|   IBIS model for TI 66ak2h06_12 DSP
[IBIS Ver]   5.0
[Disclaimer]   Please be aware that in the absence of a written agreement
|   Texas Instruments(TI) assumes no liability for:
|   (1) The accuracy of the IBIS models provided to your company,
|   however, the IBIS model is compliant to industry standard
|   IQ Level 2a.  Refer to IBIS Quality Section below for
|   for full details.
|   (2) The proper functioning of these Models in your design
|   or for any resulting applications
|   (3) Infringement of patents, copyrights or intellectual
|   property rights resulting from your use of these
|   models.
|   TI provides IBIS Models as a service to our customers and
|   therefore reserves the right to limit distribution of the
|   Models.  The information is subject to change without notice.
[File Name]  66ak2h06_12_r1p4.ibs
[File Rev]   1.4
[Date]   25 August 2014
[Source]   Texas Instruments Incorporated
[Copyright]   Property of Texas Instruments Incorporated.
|   Unauthorized reproduction and/or distribution is strictly.
|   prohibited.
|   This product is protected under copyright law and trade
|   secret law as an unpublished work.
|   Created 2012,(C) Copyright 1999-2012,
|   Texas Instruments Incorporated., All Rights Reserved.
|   These commodities are under the U.S. Government
|   distribution license control. As such,they are not to be
|   re-exported without the prior approval of the U.S.
|   Department of Commerce.
[Notes]
   For SerDes simulations use Texas Instruments IBIS AMI models
   Some IV curves contain Non monotonic data points.
|   Model Generated by R.L.L.
|   **For SerDes simulations use Texas Instruments IBIS AMI models**
|   This IBIS model also supports 66ak2h06 and 66ak2h12
|   Revision History
|   GERNERAL COMMENT: All IBIS Quality Notes below reflect latest release
|   and version of IBIS File
|   Revision 1.4 -- 25 August 2014  [Formal Updated Release]
|   -Added the [Series Pin Mapping] to assign termination.
|   Revision 1.3 -- 20 August 2014
|   -Updated the signals names to match the data manual
|   Revision 1.2 -- 23 October 2013  [Formal Updated Release]
|   -Cleaned up syntax
|   Revision 1.1 -- 22 October 2013  [Internal Release Only]
|   -Updated All DDR models
|   -Added models for DDR3L support
|   Revision 1.00--25 September 2013
|   -Formal release
|   -Updated pin names
|   Revision 0.23--29 October 2012
|   -updated device nomenclature to match new part numbering scheme
|   Revision 0.22--05 September 2012
|   -Added final packaging and clean up unused IO model selectors
|   Revision 0.21--31 August 2012
|   -Removed models not incorporated in SoC release
|   Revision 0.20--22 August 2012
|   -Added packaging details
|   Revision 0.19--22 August 2012
|   -Preliminary Model Updated
|   -Removed Pkg parasitics to test preliminary release model
|   Revision 0.18--21 August 2012
|   -Preliminary Model Updated
|   Revision 0.17--14 July 2012
|   -Preliminary Model Updated
|   Revision 0.16--14 June 2012
|   -Preliminary Model Updated
|   Revision 0.15--06 June 2012
|   -Preliminary Model Updated
|   Revision 0.14--05 June 2012
|   -Model selector added
|   Revision 0.13--30 May 2012
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[Component] 66ak2hxx
Si_location   Die
Timing_location Die
[Manufacturer] Texas Instruments
|[Package Model] 66ak2hxx
[Package]
|Variable   Typ   Min   Max
R_pkg   1.0013   0.15483   2.0653
L_pkg   2.89689nH  0.94768nH   5.3815nH
C_pkg   1.63791pF  0.87102pF   2.5609pF
[Pin] Signal_name   model_name   | Buffer Name
AM15 RSV185 NC | NC
AM11 RSV099 NC | NC
AW16 RSV161   NC | SERDES
AU16 RSV163   NC | SERDES
AV15 RSV165   NC | SERDES
AW13 RSV167   NC | SERDES
AU13 RSV169   NC | SERDES
AV12 RSV171   NC | SERDES
AW17 RSV162   NC | SERDES
AU17 RSV164   NC | SERDES
AV16 RSV166   NC | SERDES
AW14 RSV168   NC | SERDES
AU14 RSV170   NC | SERDES
AV13 RSV172   NC | SERDES
AP17 RSV173   NC | SERDES
AR16 RSV175   NC | SERDES
AT15 RSV177   NC | SERDES
AP14 RSV179   NC | SERDES
AR13 RSV181   NC | SERDES
AT12 RSV183   NC | SERDES
AP18 RSV174   NC | SERDES
AR17 RSV176   NC | SERDES
AT16 RSV178   NC | SERDES
AP15 RSV180   NC | SERDES
AR14 RSV182   NC | SERDES
AT13 RSV184   NC | SERDES
AL2 ALTCORECLKN iclkrx0p9gh | iclkrx0p9gh
AM2 ALTCORECLKP iclkrx0p9gh | iclkrx0p9gh
B37 ARMCLKN iclkrx0p9gh | iclkrx0p9gh
C37 ARMCLKP iclkrx0p9gh | iclkrx0p9gh
AF11 AVDDA1 POWER | POWER
M20 AVDDA10 POWER | POWER
Y28 AVDDA11 POWER | POWER
AB28 AVDDA12 POWER | POWER
AC28 AVDDA13 POWER | POWER
AD28 AVDDA14 POWER | POWER
AE28 AVDDA15 POWER | POWER
N20 AVDDA2 POWER | POWER
N28 AVDDA3 POWER | POWER
AH29 AVDDA4 POWER | POWER
AG26 AVDDA5 POWER | POWER
P11 AVDDA6 POWER | POWER
M13 AVDDA7 POWER | POWER
M15 AVDDA8 POWER | POWER
M18 AVDDA9 POWER | POWER
AF5 BOOTCOMPLETE bc181540h | bc181540edc50bghypbfbh
AL4 CORECLKSEL ic1815ghypbfbh | ic1815ghypbfbh
F24 CORESEL0 bc181540v | bc181540edc50bghypbfbv
E24 CORESEL1 bc181540v | bc181540edc50bghypbfbv
D24 CORESEL2 bc181540v | bc181540edc50bghypbfbv
G24 CORESEL3 bc181540v | bc181540edc50bghypbfbv
AA10 CVDD POWER | POWER
AA16 CVDD POWER | POWER
AA18 CVDD POWER | POWER
AA20 CVDD POWER | POWER
AA22 CVDD POWER | POWER
AA24 CVDD POWER | POWER
AA26 CVDD POWER | POWER
AA8 CVDD POWER | POWER
AB11 CVDD POWER | POWER
AB15 CVDD POWER | POWER
AB17 CVDD POWER | POWER
AB19 CVDD POWER | POWER
AB21 CVDD POWER | POWER
AB23 CVDD POWER | POWER
AB25 CVDD POWER | POWER
AB27 CVDD POWER | POWER
AB9 CVDD POWER | POWER
AC10 CVDD POWER | POWER
AC12 CVDD POWER | POWER
AC14 CVDD POWER | POWER
AC16 CVDD POWER | POWER
AC20 CVDD POWER | POWER
AC22 CVDD POWER | POWER
AC24 CVDD POWER | POWER
AC26 CVDD POWER | POWER
AC8 CVDD POWER | POWER
AD13 CVDD POWER | POWER
AD15 CVDD POWER | POWER
AD21 CVDD POWER | POWER
AD23 CVDD POWER | POWER
AD25 CVDD POWER | POWER
AD27 CVDD POWER | POWER
AD9 CVDD POWER | POWER
AE10 CVDD POWER | POWER
AE12 CVDD POWER | POWER
AE14 CVDD POWER | POWER
AE16 CVDD POWER | POWER
AE18 CVDD POWER | POWER
AE20 CVDD POWER | POWER
AE22 CVDD POWER | POWER
AE24 CVDD POWER | POWER
AE26 CVDD POWER | POWER
AE8 CVDD POWER | POWER
AF25 CVDD POWER | POWER
AF27 CVDD POWER | POWER
AF9 CVDD POWER | POWER
AG10 CVDD POWER | POWER
AG28 CVDD POWER | POWER
AG8 CVDD POWER | POWER
AH27 CVDD POWER | POWER
AH9 CVDD POWER | POWER
AJ10 CVDD POWER | POWER
AJ28 CVDD POWER | POWER
AJ8 CVDD POWER | POWER
AK29 CVDD POWER | POWER
AK7 CVDD POWER | POWER
AK9 CVDD POWER | POWER
AL30 CVDD POWER | POWER
AL6 CVDD POWER | POWER
AL8 CVDD POWER | POWER
AM31 CVDD POWER | POWER
AM5 CVDD POWER | POWER
L6 CVDD POWER | POWER
M25 CVDD POWER | POWER
M7 CVDD POWER | POWER
M9 CVDD POWER | POWER
N10 CVDD POWER | POWER
N12 CVDD POWER | POWER
N14 CVDD POWER | POWER
N16 CVDD POWER | POWER
N18 CVDD POWER | POWER
N22 CVDD POWER | POWER
N6 CVDD POWER | POWER
N8 CVDD POWER | POWER
P13 CVDD POWER | POWER
P15 CVDD POWER | POWER
P17 CVDD POWER | POWER
P19 CVDD POWER | POWER
P21 CVDD POWER | POWER
P27 CVDD POWER | POWER
P7 CVDD POWER | POWER
P9 CVDD POWER | POWER
R10 CVDD POWER | POWER
R12 CVDD POWER | POWER
R14 CVDD POWER | POWER
R16 CVDD POWER | POWER
R18 CVDD POWER | POWER
R20 CVDD POWER | POWER
R8 CVDD POWER | POWER
T11 CVDD POWER | POWER
T15 CVDD POWER | POWER
T17 CVDD POWER | POWER
T19 CVDD POWER | POWER
T27 CVDD POWER | POWER
T9 CVDD POWER | POWER
U10 CVDD POWER | POWER
U12 CVDD POWER | POWER
U18 CVDD POWER | POWER
U8 CVDD POWER | POWER
V15 CVDD POWER | POWER
V19 CVDD POWER | POWER
V27 CVDD POWER | POWER
V9 CVDD POWER | POWER
W10 CVDD POWER | POWER
W12 CVDD POWER | POWER
W14 CVDD POWER | POWER
W18 CVDD POWER | POWER
W20 CVDD POWER | POWER
W8 CVDD POWER | POWER
Y15 CVDD POWER | POWER
Y17 CVDD POWER | POWER
Y19 CVDD POWER | POWER
Y21 CVDD POWER | POWER
Y23 CVDD POWER | POWER
Y25 CVDD POWER | POWER
Y27 CVDD POWER | POWER
Y9 CVDD POWER | POWER
AC18 CVDD1 POWER | POWER
AD17 CVDD1 POWER | POWER
AD19 CVDD1 POWER | POWER
T13 CVDD1 POWER | POWER
T21 CVDD1 POWER | POWER
U14 CVDD1 POWER | POWER
U16 CVDD1 POWER | POWER
U20 CVDD1 POWER | POWER
V13 CVDD1 POWER | POWER
V17 CVDD1 POWER | POWER
V21 CVDD1 POWER | POWER
W16 CVDD1 POWER | POWER
AF13 VDDALV POWER | POWER
AF15 VDDALV POWER | POWER
AF17 VDDALV POWER | POWER
AF19 VDDALV POWER | POWER
AF21 VDDALV POWER | POWER
AF23 VDDALV POWER | POWER
AG12 VDDALV POWER | POWER
AG14 VDDALV POWER | POWER
AG16 VDDALV POWER | POWER
AG18 VDDALV POWER | POWER
AG20 VDDALV POWER | POWER
AG22 VDDALV POWER | POWER
AH11 VDDALV POWER | POWER
AH13 VDDALV POWER | POWER
AH15 VDDALV POWER | POWER
AH17 VDDALV POWER | POWER
AH19 VDDALV POWER | POWER
AH21 VDDALV POWER | POWER
AH23 VDDALV POWER | POWER
AH25 VDDALV POWER | POWER
AJ12 VDDALV POWER | POWER
AJ14 VDDALV POWER | POWER
AJ16 VDDALV POWER | POWER
AJ18 VDDALV POWER | POWER
AJ20 VDDALV POWER | POWER
AJ22 VDDALV POWER | POWER
AJ24 VDDALV POWER | POWER
H31 CVDD POWER | POWER
J30 CVDD POWER | POWER
K29 CVDD POWER | POWER
L28 CVDD POWER | POWER
M27 CVDD POWER | POWER
N24 CVDD POWER | POWER
N26 CVDD POWER | POWER
P23 CVDD POWER | POWER
P25 CVDD POWER | POWER
R24 CVDD POWER | POWER
R26 CVDD POWER | POWER
T23 CVDD POWER | POWER
T25 CVDD POWER | POWER
U24 CVDD POWER | POWER
U26 CVDD POWER | POWER
V23 CVDD POWER | POWER
V25 CVDD POWER | POWER
W24 CVDD POWER | POWER
W26 CVDD POWER | POWER
R22 CVDDT1 POWER | POWER
U22 CVDDT1 POWER | POWER
W22 CVDDT1 POWER | POWER
E8 DDR3AA00 ACC_OUT | SNPS_D3F_PDDRIO_NS
G9 DDR3AA01 ACC_OUT | SNPS_D3F_PDDRIO_NS
G8 DDR3AA02 ACC_OUT | SNPS_D3F_PDDRIO_NS
G10 DDR3AA03 ACC_OUT | SNPS_D3F_PDDRIO_NS
F9 DDR3AA04 ACC_OUT | SNPS_D3F_PDDRIO_NS
F8 DDR3AA05 ACC_OUT | SNPS_D3F_PDDRIO_NS
C9 DDR3AA06 ACC_OUT | SNPS_D3F_PDDRIO_NS
D9 DDR3AA07 ACC_OUT | SNPS_D3F_PDDRIO_NS
B9 DDR3AA08 ACC_OUT | SNPS_D3F_PDDRIO_NS
D8 DDR3AA09 ACC_OUT | SNPS_D3F_PDDRIO_NS
F10 DDR3AA10 ACC_OUT | SNPS_D3F_PDDRIO_NS
A9 DDR3AA11 ACC_OUT | SNPS_D3F_PDDRIO_NS
E10 DDR3AA12 ACC_OUT | SNPS_D3F_PDDRIO_NS
A10 DDR3AA13 ACC_OUT | SNPS_D3F_PDDRIO_NS
B10 DDR3AA14 ACC_OUT | SNPS_D3F_PDDRIO_NS
D10 DDR3AA15 ACC_OUT | SNPS_D3F_PDDRIO_NS
B11 DDR3ABA0 ACC_OUT | SNPS_D3F_PDDRIO_NS
C11 DDR3ABA1 ACC_OUT | SNPS_D3F_PDDRIO_NS
G11 DDR3ABA2 ACC_OUT | SNPS_D3F_PDDRIO_NS
C13 DDR3ACAS ACC_OUT | SNPS_D3F_PDDRIO_NS
A16 DDR3ACB00 DQ | SNPS_D3F_PDDRIO_NS
C15 DDR3ACB01 DQ | SNPS_D3F_PDDRIO_NS
B16 DDR3ACB02 DQ | SNPS_D3F_PDDRIO_NS
F15 DDR3ACB03 DQ | SNPS_D3F_PDDRIO_NS
D15 DDR3ACB04 DQ | SNPS_D3F_PDDRIO_NS
F14 DDR3ACB05 DQ | SNPS_D3F_PDDRIO_NS
D14 DDR3ACB06 DQ | SNPS_D3F_PDDRIO_NS
G15 DDR3ACB07 DQ | SNPS_D3F_PDDRIO_NS
D11 DDR3ACE0 ACC_OUT | SNPS_D3F_PDDRIO_NS
F11 DDR3ACE1 ACC_OUT | SNPS_D3F_PDDRIO_NS
G12 DDR3ACKE0 ACC_OUT | SNPS_D3F_PDDRIO_NS
A11 DDR3ACKE1 ACC_OUT | SNPS_D3F_PDDRIO_NS
A25 DDR3ACLKN iclkrx0p9gv | iclkrx0p9gv
B12 DDR3ACLKOUTN0 CLK_OUT | SNPS_D3F_PDDRIO_NS
B13 DDR3ACLKOUTN1 CLK_OUT | SNPS_D3F_PDDRIO_NS
A12 DDR3ACLKOUTP0 CLK_OUT | SNPS_D3F_PDDRIO_NS
A13 DDR3ACLKOUTP1 CLK_OUT | SNPS_D3F_PDDRIO_NS
B25 DDR3ACLKP iclkrx0p9gv | iclkrx0p9gv
G1 DDR3AD00 DQ | SNPS_D3F_PDDRIO_NS
H2 DDR3AD01 DQ | SNPS_D3F_PDDRIO_NS
F1 DDR3AD02 DQ | SNPS_D3F_PDDRIO_NS
G2 DDR3AD03 DQ | SNPS_D3F_PDDRIO_NS
H1 DDR3AD04 DQ | SNPS_D3F_PDDRIO_NS
E2 DDR3AD05 DQ | SNPS_D3F_PDDRIO_NS
F2 DDR3AD06 DQ | SNPS_D3F_PDDRIO_NS
D2 DDR3AD07 DQ | SNPS_D3F_PDDRIO_NS
E4 DDR3AD08 DQ | SNPS_D3F_PDDRIO_NS
F4 DDR3AD09 DQ | SNPS_D3F_PDDRIO_NS
G3 DDR3AD10 DQ | SNPS_D3F_PDDRIO_NS
A4 DDR3AD11 DQ | SNPS_D3F_PDDRIO_NS
B4 DDR3AD12 DQ | SNPS_D3F_PDDRIO_NS
H3 DDR3AD13 DQ | SNPS_D3F_PDDRIO_NS
D3 DDR3AD14 DQ | SNPS_D3F_PDDRIO_NS
D4 DDR3AD15 DQ | SNPS_D3F_PDDRIO_NS
G4 DDR3AD16 DQ | SNPS_D3F_PDDRIO_NS
H5 DDR3AD17 DQ | SNPS_D3F_PDDRIO_NS
D5 DDR3AD18 DQ | SNPS_D3F_PDDRIO_NS
F5 DDR3AD19 DQ | SNPS_D3F_PDDRIO_NS
G5 DDR3AD20 DQ | SNPS_D3F_PDDRIO_NS
D6 DDR3AD21 DQ | SNPS_D3F_PDDRIO_NS
C5 DDR3AD22 DQ | SNPS_D3F_PDDRIO_NS
B6 DDR3AD23 DQ | SNPS_D3F_PDDRIO_NS
C7 DDR3AD24 DQ | SNPS_D3F_PDDRIO_NS
F7 DDR3AD25 DQ | SNPS_D3F_PDDRIO_NS
F6 DDR3AD26 DQ | SNPS_D3F_PDDRIO_NS
A8 DDR3AD27 DQ | SNPS_D3F_PDDRIO_NS
B8 DDR3AD28 DQ | SNPS_D3F_PDDRIO_NS
G6 DDR3AD29 DQ | SNPS_D3F_PDDRIO_NS
G7 DDR3AD30 DQ | SNPS_D3F_PDDRIO_NS
D7 DDR3AD31 DQ | SNPS_D3F_PDDRIO_NS
E16 DDR3AD32 DQ | SNPS_D3F_PDDRIO_NS
G16 DDR3AD33 DQ | SNPS_D3F_PDDRIO_NS
F16 DDR3AD34 DQ | SNPS_D3F_PDDRIO_NS
G17 DDR3AD35 DQ | SNPS_D3F_PDDRIO_NS
D16 DDR3AD36 DQ | SNPS_D3F_PDDRIO_NS
D17 DDR3AD37 DQ | SNPS_D3F_PDDRIO_NS
F17 DDR3AD38 DQ | SNPS_D3F_PDDRIO_NS
E18 DDR3AD39 DQ | SNPS_D3F_PDDRIO_NS
C19 DDR3AD40 DQ | SNPS_D3F_PDDRIO_NS
D19 DDR3AD41 DQ | SNPS_D3F_PDDRIO_NS
G18 DDR3AD42 DQ | SNPS_D3F_PDDRIO_NS
F19 DDR3AD43 DQ | SNPS_D3F_PDDRIO_NS
G19 DDR3AD44 DQ | SNPS_D3F_PDDRIO_NS
B18 DDR3AD45 DQ | SNPS_D3F_PDDRIO_NS
D18 DDR3AD46 DQ | SNPS_D3F_PDDRIO_NS
F18 DDR3AD47 DQ | SNPS_D3F_PDDRIO_NS
A20 DDR3AD48 DQ | SNPS_D3F_PDDRIO_NS
B20 DDR3AD49 DQ | SNPS_D3F_PDDRIO_NS
D20 DDR3AD50 DQ | SNPS_D3F_PDDRIO_NS
G20 DDR3AD51 DQ | SNPS_D3F_PDDRIO_NS
C21 DDR3AD52 DQ | SNPS_D3F_PDDRIO_NS
E20 DDR3AD53 DQ | SNPS_D3F_PDDRIO_NS
F20 DDR3AD54 DQ | SNPS_D3F_PDDRIO_NS
G21 DDR3AD55 DQ | SNPS_D3F_PDDRIO_NS
C23 DDR3AD56 DQ | SNPS_D3F_PDDRIO_NS
G22 DDR3AD57 DQ | SNPS_D3F_PDDRIO_NS
D23 DDR3AD58 DQ | SNPS_D3F_PDDRIO_NS
F22 DDR3AD59 DQ | SNPS_D3F_PDDRIO_NS
E22 DDR3AD60 DQ | SNPS_D3F_PDDRIO_NS
B22 DDR3AD61 DQ | SNPS_D3F_PDDRIO_NS
F21 DDR3AD62 DQ | SNPS_D3F_PDDRIO_NS
D22 DDR3AD63 DQ | SNPS_D3F_PDDRIO_NS
C2 DDR3ADQM0 DM | SNPS_D3F_PDDRIO_NS
F3 DDR3ADQM1 DM | SNPS_D3F_PDDRIO_NS
A6 DDR3ADQM2 DM | SNPS_D3F_PDDRIO_NS
E6 DDR3ADQM3 DM | SNPS_D3F_PDDRIO_NS
C17 DDR3ADQM4 DM | SNPS_D3F_PDDRIO_NS
A18 DDR3ADQM5 DM | SNPS_D3F_PDDRIO_NS
D21 DDR3ADQM6 DM | SNPS_D3F_PDDRIO_NS
A22 DDR3ADQM7 DM | SNPS_D3F_PDDRIO_NS
E14 DDR3ADQM8 DM | SNPS_D3F_PDDRIO_NS
D1 DDR3ADQS0N DQS | SNPS_D3F_PDIFF_NS
E1 DDR3ADQS0P DQS | SNPS_D3F_PDIFF_NS
C3 DDR3ADQS1N DQS | SNPS_D3F_PDIFF_NS
B3 DDR3ADQS1P DQS | SNPS_D3F_PDIFF_NS
B5 DDR3ADQS2N DQS | SNPS_D3F_PDIFF_NS
A5 DDR3ADQS2P DQS | SNPS_D3F_PDIFF_NS
A7 DDR3ADQS3N DQS | SNPS_D3F_PDIFF_NS
B7 DDR3ADQS3P DQS | SNPS_D3F_PDIFF_NS
B17 DDR3ADQS4N DQS | SNPS_D3F_PDIFF_NS
A17 DDR3ADQS4P DQS | SNPS_D3F_PDIFF_NS
A19 DDR3ADQS5N DQS | SNPS_D3F_PDIFF_NS
B19 DDR3ADQS5P DQS | SNPS_D3F_PDIFF_NS
B21 DDR3ADQS6N DQS | SNPS_D3F_PDIFF_NS
A21 DDR3ADQS6P DQS | SNPS_D3F_PDIFF_NS
B23 DDR3ADQS7N DQS | SNPS_D3F_PDIFF_NS
A23 DDR3ADQS7P DQS | SNPS_D3F_PDIFF_NS
A15 DDR3ADQS8N DQS | SNPS_D3F_PDIFF_NS
B15 DDR3ADQS8P DQS | SNPS_D3F_PDIFF_NS
E12 DDR3AODT0 ACC_OUT | SNPS_D3F_PDDRIO_NS
G13 DDR3AODT1 ACC_OUT | SNPS_D3F_PDDRIO_NS
A14 DDR3ARAS ACC_OUT | SNPS_D3F_PDDRIO_NS
B14 DDR3ARESET ACC_OUT | SNPS_D3F_PDDRIO_NS
H16 DDR3ARZQ0 NC | SNPS_D3F_PZQ_NS
H10 DDR3ARZQ1 NC | SNPS_D3F_PZQ_NS
H22 DDR3ARZQ2 NC | SNPS_D3F_PZQ_NS
G14 DDR3AVREFSSTL POWER | POWER
F12 DDR3AWE ACC_OUT | SNPS_D3F_PDDRIO_NS
AA32 DDR3BA00 ACC_OUT | SNPS_D3F_PDDRIO_NS
W33 DDR3BA01 ACC_OUT | SNPS_D3F_PDDRIO_NS
W32 DDR3BA02 ACC_OUT | SNPS_D3F_PDDRIO_NS
Y34 DDR3BA03 ACC_OUT | SNPS_D3F_PDDRIO_NS
W34 DDR3BA04 ACC_OUT | SNPS_D3F_PDDRIO_NS
V34 DDR3BA05 ACC_OUT | SNPS_D3F_PDDRIO_NS
W36 DDR3BA06 ACC_OUT | SNPS_D3F_PDDRIO_NS
W37 DDR3BA07 ACC_OUT | SNPS_D3F_PDDRIO_NS
AA33 DDR3BA08 ACC_OUT | SNPS_D3F_PDDRIO_NS
Y32 DDR3BA09 ACC_OUT | SNPS_D3F_PDDRIO_NS
Y38 DDR3BA10 ACC_OUT | SNPS_D3F_PDDRIO_NS
AA39 DDR3BA11 ACC_OUT | SNPS_D3F_PDDRIO_NS
Y35 DDR3BA12 ACC_OUT | SNPS_D3F_PDDRIO_NS
Y39 DDR3BA13 ACC_OUT | SNPS_D3F_PDDRIO_NS
AA38 DDR3BA14 ACC_OUT | SNPS_D3F_PDDRIO_NS
Y36 DDR3BA15 ACC_OUT | SNPS_D3F_PDDRIO_NS
AA37 DDR3BBA0 ACC_OUT | SNPS_D3F_PDDRIO_NS
AA34 DDR3BBA1 ACC_OUT | SNPS_D3F_PDDRIO_NS
AB35 DDR3BBA2 ACC_OUT | SNPS_D3F_PDDRIO_NS
AC36 DDR3BCAS ACC_OUT | SNPS_D3F_PDDRIO_NS
AF32 DDR3BCB00 DQ | SNPS_D3F_PDDRIO_NS
AF34 DDR3BCB01 DQ | SNPS_D3F_PDDRIO_NS
AE32 DDR3BCB02 DQ | SNPS_D3F_PDDRIO_NS
AF35 DDR3BCB03 DQ | SNPS_D3F_PDDRIO_NS
AE33 DDR3BCB04 DQ | SNPS_D3F_PDDRIO_NS
AE36 DDR3BCB05 DQ | SNPS_D3F_PDDRIO_NS
AD36 DDR3BCB06 DQ | SNPS_D3F_PDDRIO_NS
AE34 DDR3BCB07 DQ | SNPS_D3F_PDDRIO_NS
AB34 DDR3BCE0 ACC_OUT | SNPS_D3F_PDDRIO_NS
AA36 DDR3BCE1 ACC_OUT | SNPS_D3F_PDDRIO_NS
AB39 DDR3BCKE0 ACC_OUT | SNPS_D3F_PDDRIO_NS
AB38 DDR3BCKE1 ACC_OUT | SNPS_D3F_PDDRIO_NS
AR39 DDR3BCLKN iclkrx0p9gv | iclkrx0p9gv
AD39 DDR3BCLKOUTN0 CLK_OUT | SNPS_D3F_PDDRIO_NS
AC38 DDR3BCLKOUTN1 CLK_OUT | SNPS_D3F_PDDRIO_NS
AD38 DDR3BCLKOUTP0 CLK_OUT | SNPS_D3F_PDDRIO_NS
AC39 DDR3BCLKOUTP1 CLK_OUT | SNPS_D3F_PDDRIO_NS
AR38 DDR3BCLKP iclkrx0p9gv | iclkrx0p9gv
L38 DDR3BD00 DQ | SNPS_D3F_PDDRIO_NS
N34 DDR3BD01 DQ | SNPS_D3F_PDDRIO_NS
M37 DDR3BD02 DQ | SNPS_D3F_PDDRIO_NS
L39 DDR3BD03 DQ | SNPS_D3F_PDDRIO_NS
N33 DDR3BD04 DQ | SNPS_D3F_PDDRIO_NS
N37 DDR3BD05 DQ | SNPS_D3F_PDDRIO_NS
N36 DDR3BD06 DQ | SNPS_D3F_PDDRIO_NS
N38 DDR3BD07 DQ | SNPS_D3F_PDDRIO_NS
T32 DDR3BD08 DQ | SNPS_D3F_PDDRIO_NS
R32 DDR3BD09 DQ | SNPS_D3F_PDDRIO_NS
P35 DDR3BD10 DQ | SNPS_D3F_PDDRIO_NS
R39 DDR3BD11 DQ | SNPS_D3F_PDDRIO_NS
R38 DDR3BD12 DQ | SNPS_D3F_PDDRIO_NS
N32 DDR3BD13 DQ | SNPS_D3F_PDDRIO_NS
R33 DDR3BD14 DQ | SNPS_D3F_PDDRIO_NS
P36 DDR3BD15 DQ | SNPS_D3F_PDDRIO_NS
T34 DDR3BD16 DQ | SNPS_D3F_PDDRIO_NS
R34 DDR3BD17 DQ | SNPS_D3F_PDDRIO_NS
T35 DDR3BD18 DQ | SNPS_D3F_PDDRIO_NS
R37 DDR3BD19 DQ | SNPS_D3F_PDDRIO_NS
R36 DDR3BD20 DQ | SNPS_D3F_PDDRIO_NS
U37 DDR3BD21 DQ | SNPS_D3F_PDDRIO_NS
T36 DDR3BD22 DQ | SNPS_D3F_PDDRIO_NS
U38 DDR3BD23 DQ | SNPS_D3F_PDDRIO_NS
V35 DDR3BD24 DQ | SNPS_D3F_PDDRIO_NS
U36 DDR3BD25 DQ | SNPS_D3F_PDDRIO_NS
U34 DDR3BD26 DQ | SNPS_D3F_PDDRIO_NS
W38 DDR3BD27 DQ | SNPS_D3F_PDDRIO_NS
W39 DDR3BD28 DQ | SNPS_D3F_PDDRIO_NS
U33 DDR3BD29 DQ | SNPS_D3F_PDDRIO_NS
V32 DDR3BD30 DQ | SNPS_D3F_PDDRIO_NS
V36 DDR3BD31 DQ | SNPS_D3F_PDDRIO_NS
AG37 DDR3BD32 DQ | SNPS_D3F_PDDRIO_NS
AF36 DDR3BD33 DQ | SNPS_D3F_PDDRIO_NS
AG38 DDR3BD34 DQ | SNPS_D3F_PDDRIO_NS
AG34 DDR3BD35 DQ | SNPS_D3F_PDDRIO_NS
AG36 DDR3BD36 DQ | SNPS_D3F_PDDRIO_NS
AH34 DDR3BD37 DQ | SNPS_D3F_PDDRIO_NS
AH35 DDR3BD38 DQ | SNPS_D3F_PDDRIO_NS
AG32 DDR3BD39 DQ | SNPS_D3F_PDDRIO_NS
AH32 DDR3BD40 DQ | SNPS_D3F_PDDRIO_NS
AJ33 DDR3BD41 DQ | SNPS_D3F_PDDRIO_NS
AH36 DDR3BD42 DQ | SNPS_D3F_PDDRIO_NS
AJ34 DDR3BD43 DQ | SNPS_D3F_PDDRIO_NS
AJ36 DDR3BD44 DQ | SNPS_D3F_PDDRIO_NS
AH39 DDR3BD45 DQ | SNPS_D3F_PDDRIO_NS
AH38 DDR3BD46 DQ | SNPS_D3F_PDDRIO_NS
AJ37 DDR3BD47 DQ | SNPS_D3F_PDDRIO_NS
AK39 DDR3BD48 DQ | SNPS_D3F_PDDRIO_NS
AK38 DDR3BD49 DQ | SNPS_D3F_PDDRIO_NS
AK36 DDR3BD50 DQ | SNPS_D3F_PDDRIO_NS
AK35 DDR3BD51 DQ | SNPS_D3F_PDDRIO_NS
AL34 DDR3BD52 DQ | SNPS_D3F_PDDRIO_NS
AL36 DDR3BD53 DQ | SNPS_D3F_PDDRIO_NS
AL37 DDR3BD54 DQ | SNPS_D3F_PDDRIO_NS
AL33 DDR3BD55 DQ | SNPS_D3F_PDDRIO_NS
AN34 DDR3BD56 DQ | SNPS_D3F_PDDRIO_NS
AN36 DDR3BD57 DQ | SNPS_D3F_PDDRIO_NS
AN33 DDR3BD58 DQ | SNPS_D3F_PDDRIO_NS
AM34 DDR3BD59 DQ | SNPS_D3F_PDDRIO_NS
AM35 DDR3BD60 DQ | SNPS_D3F_PDDRIO_NS
AM38 DDR3BD61 DQ | SNPS_D3F_PDDRIO_NS
AM36 DDR3BD62 DQ | SNPS_D3F_PDDRIO_NS
AN37 DDR3BD63 DQ | SNPS_D3F_PDDRIO_NS
N39 DDR3BDQM0 DM | SNPS_D3F_PDDRIO_NS
P34 DDR3BDQM1 DM | SNPS_D3F_PDDRIO_NS
U39 DDR3BDQM2 DM | SNPS_D3F_PDDRIO_NS
U32 DDR3BDQM3 DM | SNPS_D3F_PDDRIO_NS
AG33 DDR3BDQM4 DM | SNPS_D3F_PDDRIO_NS
AG39 DDR3BDQM5 DM | SNPS_D3F_PDDRIO_NS
AK34 DDR3BDQM6 DM | SNPS_D3F_PDDRIO_NS
AM39 DDR3BDQM7 DM | SNPS_D3F_PDDRIO_NS
AE37 DDR3BDQM8 DM | SNPS_D3F_PDDRIO_NS
M39 DDR3BDQS0N DQS | SNPS_D3F_PDIFF_NS
M38 DDR3BDQS0P DQS | SNPS_D3F_PDIFF_NS
P38 DDR3BDQS1N DQS | SNPS_D3F_PDIFF_NS
P39 DDR3BDQS1P DQS | SNPS_D3F_PDIFF_NS
T38 DDR3BDQS2N DQS | SNPS_D3F_PDIFF_NS
T39 DDR3BDQS2P DQS | SNPS_D3F_PDIFF_NS
V38 DDR3BDQS3N DQS | SNPS_D3F_PDIFF_NS
V39 DDR3BDQS3P DQS | SNPS_D3F_PDIFF_NS
AF39 DDR3BDQS4N DQS | SNPS_D3F_PDIFF_NS
AF38 DDR3BDQS4P DQS | SNPS_D3F_PDIFF_NS
AJ38 DDR3BDQS5N DQS | SNPS_D3F_PDIFF_NS
AJ39 DDR3BDQS5P DQS | SNPS_D3F_PDIFF_NS
AL38 DDR3BDQS6N DQS | SNPS_D3F_PDIFF_NS
AL39 DDR3BDQS6P DQS | SNPS_D3F_PDIFF_NS
AN39 DDR3BDQS7N DQS | SNPS_D3F_PDIFF_NS
AN38 DDR3BDQS7P DQS | SNPS_D3F_PDIFF_NS
AE38 DDR3BDQS8N DQS | SNPS_D3F_PDIFF_NS
AE39 DDR3BDQS8P DQS | SNPS_D3F_PDIFF_NS
AC33 DDR3BODT0 ACC_OUT   | SNPS_D3F_PDDRIO_NS
AD34 DDR3BODT1 ACC_OUT   | SNPS_D3F_PDDRIO_NS
AD32 DDR3BRAS ACC_OUT   | SNPS_D3F_PDDRIO_NS
AC32 DDR3BRESET ACC_OUT | SNPS_D3F_PDDRIO_NS
AA31 DDR3BRZQ0 NC | SNPS_D3F_PZQ_NS
P32 DDR3BRZQ1 NC  | SNPS_D3F_PZQ_NS
AK32 DDR3BRZQ2 NC | SNPS_D3F_PZQ_NS
AC31 DDR3BVREFSSTL POWER | POWER
AC37 DDR3BWE ACC_OUT | SNPS_D3F_PDDRIO_NS
AA28 DVDD15 POWER | POWER
AA30 DVDD15 POWER | POWER
AB29 DVDD15 POWER | POWER
AB31 DVDD15 POWER | POWER
AC30 DVDD15 POWER | POWER
AD29 DVDD15 POWER | POWER
AD31 DVDD15 POWER | POWER
AE30 DVDD15 POWER | POWER
AF29 DVDD15 POWER | POWER
AF31 DVDD15 POWER | POWER
AG30 DVDD15 POWER | POWER
AH31 DVDD15 POWER | POWER
AJ30 DVDD15 POWER | POWER
AK31 DVDD15 POWER | POWER
AL32 DVDD15 POWER | POWER
H11 DVDD15 POWER  | POWER
H13 DVDD15 POWER  | POWER
H15 DVDD15 POWER  | POWER
H17 DVDD15 POWER  | POWER
H19 DVDD15 POWER  | POWER
H21 DVDD15 POWER  | POWER
H23 DVDD15 POWER  | POWER
H7 DVDD15 POWER   | POWER
H9 DVDD15 POWER   | POWER
J10 DVDD15 POWER | POWER
J12 DVDD15 POWER | POWER
J14 DVDD15 POWER | POWER
J16 DVDD15 POWER | POWER
J18 DVDD15 POWER | POWER
J20 DVDD15 POWER | POWER
J22 DVDD15 POWER | POWER
J6 DVDD15 POWER  | POWER
J8 DVDD15 POWER  | POWER
K11 DVDD15 POWER | POWER
K13 DVDD15 POWER | POWER
K15 DVDD15 POWER | POWER
K17 DVDD15 POWER | POWER
K19 DVDD15 POWER | POWER
K21 DVDD15 POWER | POWER
K23 DVDD15 POWER | POWER
K7 DVDD15 POWER  | POWER
K9 DVDD15 POWER  | POWER
L10 DVDD15 POWER | POWER
L12 DVDD15 POWER | POWER
L14 DVDD15 POWER | POWER
L16 DVDD15 POWER | POWER
L18 DVDD15 POWER | POWER
L20 DVDD15 POWER | POWER
L32 DVDD15 POWER | POWER
L8 DVDD15 POWER  | POWER
M11 DVDD15 POWER | POWER
M17 DVDD15 POWER | POWER
M19 DVDD15 POWER | POWER
M31 DVDD15 POWER | POWER
P29 DVDD15 POWER | POWER
P31 DVDD15 POWER | POWER
R28 DVDD15 POWER | POWER
R30 DVDD15 POWER | POWER
T29 DVDD15 POWER | POWER
T31 DVDD15 POWER | POWER
U28 DVDD15 POWER | POWER
U30 DVDD15 POWER | POWER
V29 DVDD15 POWER | POWER
V31 DVDD15 POWER | POWER
W28 DVDD15 POWER | POWER
W30 DVDD15 POWER | POWER
Y29 DVDD15 POWER | POWER
Y31 DVDD15 POWER | POWER
AA6 DVDD18 POWER | POWER
AB5 DVDD18 POWER | POWER
AB7 DVDD18 POWER | POWER
AC6 DVDD18 POWER | POWER
AD7 DVDD18 POWER | POWER
AE6 DVDD18 POWER | POWER
AF7 DVDD18 POWER | POWER
AG6 DVDD18 POWER | POWER
AJ26 DVDD18 POWER | POWER
AK27 DVDD18 POWER | POWER
AL26 DVDD18 POWER | POWER
AL28 DVDD18 POWER | POWER
AM27 DVDD18 POWER | POWER
AM29 DVDD18 POWER | POWER
H25 DVDD18 POWER  | POWER
H27 DVDD18 POWER  | POWER
J26 DVDD18 POWER  | POWER
J28 DVDD18 POWER  | POWER
J32 DVDD18 POWER  | POWER
K25 DVDD18 POWER  | POWER
K27 DVDD18 POWER  | POWER
K31 DVDD18 POWER  | POWER
L24 DVDD18 POWER  | POWER
L26 DVDD18 POWER  | POWER
L30 DVDD18 POWER  | POWER
M29 DVDD18 POWER  | POWER
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|********************  DIFF PIN  *******************************
[Diff_pin]   inv_pin vdiff tdelay_typ   tdelay_min  tdelay_max
E1   D1   200mV   NA  NA  NA  || DDR3ADQS0P & DDR3ADQS0N
B3   C3   200mV   NA  NA  NA  || DDR3ADQS1P & DDR3ADQS1N
A5   B5   200mV   NA  NA  NA  || DDR3ADQS2P & DDR3ADQS2N
B7   A7   200mV   NA  NA  NA  || DDR3ADQS3P & DDR3ADQS3N
A17   B17   200mV   NA  NA  NA  || DDR3ADQS4P & DDR3ADQS4N
B19   A19   200mV   NA  NA  NA  || DDR3ADQS5P & DDR3ADQS5N
A21   B21   200mV   NA  NA  NA  || DDR3ADQS6P & DDR3ADQS6N
A23   B23   200mV   NA  NA  NA  || DDR3ADQS7P & DDR3ADQS7N
B15   A15   200mV   NA  NA  NA  || DDR3ADQS8P & DDR3ADQS8N
M38   M39   200mV   NA  NA  NA  || DDR3BDQS0P & DDR3BDQS0N
P39   P38   200mV   NA  NA  NA  || DDR3BDQS1P & DDR3BDQS1N
T39   T38   200mV   NA  NA  NA  || DDR3BDQS2P & DDR3BDQS2N
V39   V38   200mV   NA  NA  NA  || DDR3BDQS3P & DDR3BDQS3N
AF38   AF39   200mV   NA  NA  NA  || DDR3BDQS4P & DDR3BDQS4N
AJ39   AJ38   200mV   NA  NA  NA  || DDR3BDQS5P & DDR3BDQS5N
AL39   AL38   200mV   NA  NA  NA  || DDR3BDQS6P & DDR3BDQS6N
AN38   AN39   200mV   NA  NA  NA  || DDR3BDQS7P & DDR3BDQS7N
AE39   AE38   200mV   NA  NA  NA  || DDR3BDQS8P & DDR3BDQS8N
AL3   AK3   NA   NA  NA  NA  || SYSCLKP & SYSCLKN
AM2   AL2   NA   NA  NA  NA  || ALTCORECLKP & ALTCORECLKN
C37   B37   NA   NA  NA  NA  || ARMCLKP & ARMCLKN
B25   A25   NA   NA  NA  NA  || DDR3ACLKP & DDR3ACLKN
AR38   AR39   NA   NA  NA  NA  || DDR3BCLKP & DDR3BCLKN
AV33   AV34   NA   NA  NA  NA  || PASSCLKP & PASSCLKN
AW31   AW32   NA   NA  NA  NA  || PCIECLKP & PCIECLKN
AW34   AW35   NA   NA  NA  NA  || SRIOSGMIICLKP & SRIOSGMIICLKN
AM1   AL1   NA   NA  NA  NA  || TSREFCLKP & TSREFCLKN
AR2   AP2   NA   NA  NA  NA  || RSV186 & RSV187
AN1   AP1   NA   NA  NA  NA  || TSRXCLKOUT0P & TSRXCLKOUT0N
AN3   AP3   NA   NA  NA  NA  || TSRXCLKOUT1P & TSRXCLKOUT1N
[Series Pin Mapping]   pin_2   model_name
AL2   AM2   s_iclkrx0p9gh   || ALTCORECLKN/P
B37   C37   s_iclkrx0p9gh   || ARMCLKN/P
AK3   AL3   s_iclkrx0p9gh   || SYSCLKN/P
A25   B25   s_iclkrx0p9gv   || DDR3ACLKN/P
AR39   AR38   s_iclkrx0p9gv   || DDR3BCLKN/P
AV34   AV33   s_iclkrx0p9gv   || PASSCLKN/P
AW32   AW31   s_iclkrx0p9gv   || PCIECLKN/P
AW35   AW34   s_iclkrx0p9gv   || SRIOSGMIICLKN/P
|---------------- DDR CLK_OUT IBIS Model -------------------
[Model Selector]   CLK_OUT
|pddrio.ibs   [18 October 2013 revision 0.1]
|renamed PDDRIO_D3FP3_
| ----------- DDR3 CLK_OUT Output Model Selector -----------
PDDRIO_D3FP3_34   DDR3 D3F_PDDRIO cell  Z0=34-Ohm
PDDRIO_D3FP3_40   DDR3 D3F_PDDRIO cell  Z0=40-Ohm
PDDRIO_D3FP3_48   DDR3 D3F_PDDRIO cell  Z0=48-Ohm
| ---------- DDR3L CLK_OUT Output Model Selector -----------
PDDRIO_D3FP3L_34   DDR3L D3F_PDDRIO cell  Z0=34-Ohm
PDDRIO_D3FP3L_40   DDR3L D3F_PDDRIO cell  Z0=40-Ohm
PDDRIO_D3FP3L_48   DDR3L D3F_PDDRIO cell  Z0=48-Ohm
|---------------- DDR ACC_OUT IBIS Model -------------------
[Model Selector]   ACC_OUT
|pddrio.ibs   [18 October 2013 revision 0.1]
|renamed PDDRIO_D3FP3_
| ---------- DDR3 ACC_OUT Output Model Selector ------------
PDDRIO_D3FP3_34   DDR3 D3F_PDDRIO cell  Z0=34-Ohm
PDDRIO_D3FP3_40   DDR3 D3F_PDDRIO cell  Z0=40-Ohm
PDDRIO_D3FP3_48   DDR3 D3F_PDDRIO cell  Z0=48-Ohm
| --------- DDR3L ACC_OUT Output Model Selector ------------
PDDRIO_D3FP3L_34   DDR3L D3F_PDDRIO cell  Z0=34-Ohm
PDDRIO_D3FP3L_40   DDR3L D3F_PDDRIO cell  Z0=40-Ohm
PDDRIO_D3FP3L_48   DDR3L D3F_PDDRIO cell  Z0=48-Ohm
|---------------- DDR DM IBIS Model -------------------
[Model Selector]   DM
|pddrio.ibs   [18 October 2013 revision 0.1]
|renamed PDDRIO_D3FP3_
| ------------- DDR3 DM Output Model Selector --------------
PDDRIO_D3FP3_34   DDR3 D3F_PDDRIO cell  Z0=34-Ohm
PDDRIO_D3FP3_40   DDR3 D3F_PDDRIO cell  Z0=40-Ohm
PDDRIO_D3FP3_48   DDR3 D3F_PDDRIO cell  Z0=48-Ohm
| ------------ DDR3L DM Output Model Selector --------------
PDDRIO_D3FP3L_34   DDR3L D3F_PDDRIO cell  Z0=34-Ohm
PDDRIO_D3FP3L_40   DDR3L D3F_PDDRIO cell  Z0=40-Ohm
PDDRIO_D3FP3L_48   DDR3L D3F_PDDRIO cell  Z0=48-Ohm
| -------------- DDR3 DM Input Model Selector --------------
PDDRIO_D3FP3_ODT120   DDR3 D3F_PDDRIO cell 120-Ohm ODT Receiver
PDDRIO_D3FP3_ODT40   DDR3 D3F_PDDRIO cell 40-Ohm ODT Receiver
PDDRIO_D3FP3_ODT60   DDR3 D3F_PDDRIO cell 60-Ohm ODT Receiver
PDDRIO_D3FP3_ODTOFF   DDR3 D3F_PDDRIO cell ODT off Receiver
| ------------- DDR3L DM Input Model Selector --------------
PDDRIO_D3FP3L_ODT120   DDR3L D3F_PDDRIO cell 120-Ohm ODT Receiver
PDDRIO_D3FP3L_ODT40   DDR3L D3F_PDDRIO cell 40-Ohm ODT Receiver
PDDRIO_D3FP3L_ODT60   DDR3L D3F_PDDRIO cell 60-Ohm ODT Receiver
PDDRIO_D3FP3L_ODTOFF   DDR3L D3F_PDDRIO cell ODT off Receiver
|---------------- DDR DQ IBIS Model -------------------
[Model Selector]   DQ
|pddrio.ibs   [18 October 2013 revision 0.1]
|renamed PDDRIO_D3FP3_
| -------------- DDR3 DQ Output Model Selector --------------
PDDRIO_D3FP3_34   DDR3 D3F_PDDRIO cell  Z0=34-Ohm
PDDRIO_D3FP3_40   DDR3 D3F_PDDRIO cell  Z0=40-Ohm
PDDRIO_D3FP3_48   DDR3 D3F_PDDRIO cell  Z0=48-Ohm
| ------------- DDR3L DQ Output Model Selector --------------
PDDRIO_D3FP3L_34   DDR3L D3F_PDDRIO cell  Z0=34-Ohm
PDDRIO_D3FP3L_40   DDR3L D3F_PDDRIO cell  Z0=40-Ohm
PDDRIO_D3FP3L_48   DDR3L D3F_PDDRIO cell  Z0=48-Ohm
| --------------- DDR3 DQ Input Model Selector --------------
PDDRIO_D3FP3_ODT120   DDR3 D3F_PDDRIO cell 120-Ohm ODT Receiver
PDDRIO_D3FP3_ODT40   DDR3 D3F_PDDRIO cell 40-Ohm ODT Receiver
PDDRIO_D3FP3_ODT60   DDR3 D3F_PDDRIO cell 60-Ohm ODT Receiver
PDDRIO_D3FP3_ODTOFF   DDR3 D3F_PDDRIO cell ODT off Receiver
| -------------- DDR3L DQ Input Model Selector --------------
PDDRIO_D3FP3L_ODT120   DDR3L D3F_PDDRIO cell 120-Ohm ODT Receiver
PDDRIO_D3FP3L_ODT40   DDR3L D3F_PDDRIO cell 40-Ohm ODT Receiver
PDDRIO_D3FP3L_ODT60   DDR3L D3F_PDDRIO cell 60-Ohm ODT Receiver
PDDRIO_D3FP3L_ODTOFF   DDR3L D3F_PDDRIO cell ODT off Receiver
| ----------------- DDR DQS IBIS Model --------------------
[Model Selector]   DQS
|pdiff.ibs   [18 October 2013 revision 0.1]
|renamed PDIFF_D3FP3_
| -------------- DDR3 DQS Input Model Selector ------------
PDIFF_D3FF3_ODT120   DDR3 D3F_PDIFF cell 120-Ohm ODT Receiver
PDIFF_D3FF3_ODT40   DDR3 D3F_PDIFF cell 40-Ohm ODT Receiver
PDIFF_D3FF3_ODT60   DDR3 D3F_PDIFF cell 60-Ohm ODT Receiver
PDIFF_D3FF3_ODTOFF   DDR3 D3F_PDIFF cell ODT off Receiver
| -------------- DDR3L DQS Input Model Selector ------------
PDIFF_D3FF3L_ODT120   DDR3L D3F_PDIFF cell 120-Ohm ODT Receiver
PDIFF_D3FF3L_ODT40   DDR3L D3F_PDIFF cell 40-Ohm ODT Receiver
PDIFF_D3FF3L_ODT60   DDR3L D3F_PDIFF cell 60-Ohm ODT Receiver
PDIFF_D3FF3L_ODTOFF   DDR3L D3F_PDIFF cell ODT off Receiver
| -------------- DDR3 DQS Output Model Selector ------------
PDIFF_D3FF3_34   DDR3 D3F_PDIFF cell  Z0=34-Ohm
PDIFF_D3FF3_40   DDR3 D3F_PDIFF cell  Z0=40-Ohm
PDIFF_D3FF3_48   DDR3 D3F_PDIFF cell  Z0=48-Ohm
| -------------- DDR3L DQS Output Model Selector -----------
PDIFF_D3FF3L_34   DDR3L D3F_PDIFF cell  Z0=34-Ohm
PDIFF_D3FF3L_40   DDR3L D3F_PDIFF cell  Z0=40-Ohm
PDIFF_D3FF3L_48   DDR3L D3F_PDIFF cell  Z0=48-Ohm
|----------------  iclkrx0p9gh IBIS Model --------------
[Model Selector]   iclkrx0p9gh
|iclkrx0p9gh_encmint_0.ibs   [12Feb12 revision 2.0]
|iclkrx0p9gh_encmint_1.ibs   [12Feb12 revision 2.0]
iclkrx0p9gh_encmint_0   Ext. CommMode Used
| When set to zero external common mode used
iclkrx0p9gh_encmint_1   Int. CommMode Used
| When set to one internal common mode used
|----------------  iclkrx0p9gv IBIS Model ---------------
[Model Selector]   iclkrx0p9gv
|iclkrx0p9gv_encmint_0.ibs   [12Feb12 revision 2.0]
|iclkrx0p9gv_encmint_1.ibs   [12Feb12 revision 2.0]
iclkrx0p9gv_encmint_0   Ext. CommMode Used
| When set to zero external common mode used
iclkrx0p9gv_encmint_1   Int. CommMode Used
| When set to one internal common mode used
|----------------  s_iclkrx0p9gh IBIS Model ---------------
[Model Selector]  s_iclkrx0p9gh
s_iclkrx0p9gh_encmint_0   Ext. CommMode Used
s_iclkrx0p9gh_encmint_1   Int. CommMode Used
|----------------  s_iclkrx0p9gv IBIS Model ---------------
[Model Selector]  s_iclkrx0p9gv
s_iclkrx0p9gv_encmint_0   Ext. CommMode Used
s_iclkrx0p9gv_encmint_1   Int. CommMode Used
|----------------  D3F_PZQ_NS IBIS Model -----------
|D3F_PZQ_NS.ibs
|place holder for termination IO buffers
|--------bc181540edc50bghypbfbh IBIS Model -----------
[Model Selector]   bc181540h
|bc181540edc50bghypbfbh.ibs   [23Jan12 revision 1.0]
bc181540h_40CCLASS_1P8  Cell operated at 1.8(nom)
|40CCLASS_1P8; 40C:130MHZ@5PF CLASS IO MODE
bc181540h_WK_PD_ON_1P8  Cell operated at 1.8(nom)
|WK_PD_ON_1P8; INPUT MODE WITH WK_PD_ON
bc181540h_40ECLASS_1P8  Cell operated at 1.8(nom)
|40ECLASS_1P8; 40E:230MHZ@5PF CLASS IO MODE
bc181540h_WK_PU_ON_1P8  Cell operated at 1.8(nom)
|WK_PU_ON_1P8; INPUT MODE WITH WK_PU_ON
bc181540h_40DCLASS_1P8  Cell operated at 1.8(nom)
|40DCLASS_1P8; 40D:200MHZ@5PF CLASS IO MODE
bc181540h_50BCLASS_1P8  Cell operated at 1.8(nom)
|50BCLASS_1P8; 50B:100MHZ@5PF CLASS IO MODE
|------ bc181540edc50bghypbfbv IBIS Model --------
[Model Selector]   bc181540v
|bc181540edc50bghypbfbv.ibs  [23Jan12 revision 1.0]
bc181540v_40CCLASS_1P5  Cell operated at 1.5(nom)
|40CCLASS_1P5; 40C:130MHZ@5PF CLASS IO MODE
bc181540v_WK_PD_ON_1P5  Cell operated at 1.5(nom)
|WK_PD_ON_1P5; INPUT MODE WITH WK_PD_ON
bc181540v_40ECLASS_1P5  Cell operated at 1.5(nom)
|40ECLASS_1P5; 40E:230MHZ@5PF CLASS IO MODE
bc181540v_WK_PU_ON_1P5  Cell operated at 1.5(nom)
|WK_PU_ON_1P5; INPUT MODE WITH WK_PU_ON
bc181540v_40DCLASS_1P5  Cell operated at 1.5(nom)
|40DCLASS_1P5; 40D:200MHZ@5PF CLASS IO MODE
bc181540v_50BCLASS_1P5  Cell operated at 1.5(nom)
|50BCLASS_1P5; 50B:100MHZ@5PF CLASS IO MODE
bc181540v_40CCLASS_1P8  Cell operated at 1.8(nom)
|40CCLASS_1P8; 40C:130MHZ@5PF CLASS IO MODE
bc181540v_WK_PD_ON_1P8  Cell operated at 1.8(nom)
|WK_PD_ON_1P8; INPUT MODE WITH WK_PD_ON
bc181540v_40ECLASS_1P8  Cell operated at 1.8(nom)
|40ECLASS_1P8; 40E:230MHZ@5PF CLASS IO MODE
bc181540v_WK_PU_ON_1P8  Cell operated at 1.8(nom)
|WK_PU_ON_1P8; INPUT MODE WITH WK_PU_ON
bc181540v_40DCLASS_1P8  Cell operated at 1.8(nom)
|40DCLASS_1P8; 40D:200MHZ@5PF CLASS IO MODE
bc181540v_50BCLASS_1P8  Cell operated at 1.8(nom)
|50BCLASS_1P8; 50B:100MHZ@5PF CLASS IO MODE
|--------bi2c1815gfzhsh IBIS Model ----------
[Model Selector]   bi2c1815gfzhsh
|bi2c1815gfzhsh.ibs   [11Jan12 revision 1.0]
bi2c1815h_HS_SLAVE_MODE_1P8  Cell operated at 1.8(nom)
|HS_SLAVE_MODE_1P8; I2C HS SLAVE MODE
bi2c1815h_FAST_STD_1P8  Cell operated at 1.8(nom)
|FAST_STD_1P8; I2C FAST AND STD MODE
bi2c1815h_HS_MASTER_MODE_1P8  Cell operated at 1.8(nom)
|HS_MASTER_MODE_1P8; I2C HS MASTER MODE
|--------- bi2c1815gfzhsv IBIS Model ------------
[Model Selector] bi2c1815gfzhsv
|bi2c1815gfzhsv.ibs   [11Jan12 revision 1.0]
bi2c1815v_HS_SLAVE_MODE_1P8  Cell operated at 1.8(nom)
|HS_SLAVE_MODE_1P8; I2C HS SLAVE MODE
bi2c1815v_FAST_STD_1P8  Cell operated at 1.8(nom)
|FAST_STD_1P8; I2C FAST AND STD MODE
bi2c1815v_HS_MASTER_MODE_1P8  Cell operated at 1.8(nom)
|HS_MASTER_MODE_1P8; I2C HS MASTER MODE
|------- ic1815ghypbfbh IBIS Model ------------
[Model Selector] ic1815ghypbfbh
|ic1815ghypbfbh.ibs   [27Dec11 revision 1.0]
ic1815h_WK_PD_ON_1P8  Cell operated at 1.8(nom)
|WK_PD_ON_1P8; WK_PD_ON
ic1815h_WK_PU_ON_1P8  Cell operated at 1.8(nom)
|WK_PU_ON_1P8; WK_PU_ON
ic1815h_RX_MODE_1P8  Cell operated at 1.8(nom)
|RX_MODE_1P8
|---------------- ic1815ghypbfbv IBIS Model --------
[Model Selector] ic1815ghypbfbv
|ic1815ghypbfbv.ibs   [27Dec11 revision 1.0]
ic1815v_WK_PD_ON_1P8  Cell operated at 1.8(nom)
|WK_PD_ON_1P8; WK_PD_ON
ic1815v_WK_PU_ON_1P8  Cell operated at 1.8(nom)
|WK_PU_ON_1P8; WK_PU_ON
ic1815v_RX_MODE_1P8  Cell operated at 1.8(nom)
|RX_MODE_1P8
|---------------- olvds18gh IBIS Model -----------
[Model Selector] olvds18gh
|olvds18gh.ibs   [30Dec11 revision 1.0]
OLVDS18GH_SUBLVDS_MODE_3MA_100_1P8  Cell operated at 1.8(nom)
|SUBLVDS MODE :3MA OUTPUT CURRENT SETTING WITH 100 OHM INT. TERM.
OLVDS18GH_2MA_200_1P8  Cell operated at 1.8(nom)
|2MA OUTPUT CURRENT SETTING WITH 200 OHM INT. TERM.
OLVDS18GH_4MA_100_1P8  Cell operated at 1.8(nom)
|4MA OUTPUT CURRENT SETTING WITH 100 OHM INT. TERM.
OLVDS18GH_SUBLVDS_MODE_2.5MA_100_1P8  Cell operated at 1.8(nom)
|SUBLVDS MODE : 2.5MA OUTPUT CURRENT SETTING WITH 100 OHM INT. TERM.
OLVDS18GH_3.5MA_100_1P8  Cell operated at 1.8(nom)
|3.5MA OUTPUT CURRENT SETTING WITH 100 OHM INT. TERM.
OLVDS18GH_SUBLVDS_MODE_2.66MA_200_1P8  Cell operated at 1.8(nom)
|SUBLVDS MODE :2.66MA OUTPUT CURRENT SETTING WITH 200 OHM INT. TERM.
OLVDS18GH_SUBLVDS_MODE_2MA_200_1P8  Cell operated at 1.8(nom)
|SUBLVDS MODE :2MA OUTPUT CURRENT SETTING WITH 200 OHM INT. TERM.
OLVDS18GH_4MA_200_1P8  Cell operated at 1.8(nom)
|4MA OUTPUT CURRENT SETTING WITH 200 OHM INT. TERM.
OLVDS18GH_3.33MA_200_1P8  Cell operated at 1.8(nom)
|3.33MA OUTPUT CURRENT SETTING WITH 200 OHM INT. TERM.
OLVDS18GH_SUBLVDS_MODE_4MA_100_1P8  Cell operated at 1.8(nom)
|SUBLVDS MODE :4MA OUTPUT CURRENT SETTING WITH 100 OHM INT. TERM.
OLVDS18GH_SUBLVDS_MODE_3.5MA_100_1P8  Cell operated at 1.8(nom)
|SUBLVDS MODE :3.5MA OUTPUT CURRENT SETTING WITH 100 OHM INT. TERM.
OLVDS18GH_3MA_100_1P8  Cell operated at 1.8(nom)
|3MA OUTPUT CURRENT SETTING WITH 100 OHM INT. TERM.
OLVDS18GH_SUBLVDS_MODE_4MA_200_1P8  Cell operated at 1.8(nom)
|SUBLVDS MODE :4MA OUTPUT CURRENT SETTING WITH 200 OHM INT. TERM.
OLVDS18GH_2.5MA_100_1P8  Cell operated at 1.8(nom)
|2.5MA OUTPUT CURRENT SETTING WITH 100 OHM INT. TERM.
OLVDS18GH_SUBLVDS_MODE_3.33MA_200_1P8  Cell operated at 1.8(nom)
|SUBLVDS MODE :3.33MA OUTPUT CURRENT SETTING WITH 200 OHM INT. TERM.
OLVDS18GH_2.66MA_200_1P8  Cell operated at 1.8(nom)
|   Package Model Definition
[Define Package Model]  66ak2hxx
[Manufacturer]   Texas Instruments Incorporated
[OEM]   Texas Instruments Incorporated
[Description]   66ak2hxx pkg with all signals except AMI
|   file: pgz0877ar-e8_080212
|   file dated: August 30, 2012
[Number Of Pins]   665
[Pin Numbers]
AM16 | 1 BGA-AM16 RSV024
AN16 | 2 BGA-AN16 RSV068
AM15 | 3 BGA-AM15 RSV185
AM14 | 4 BGA-AM14 RSV025
AM11 | 5 BGA-AM11 RSV099
AN10 | 6 BGA-AN10 RSV019
AM9  | 7 BGA-AM9 HYP0REFRES
AW16 | 8 BGA-AW16 RSV161
AW17 | 9 BGA-AW17 RSV162
AV18 | 10 BGA-AV18 RSV061
AU16 | 11 BGA-AU16 RSV163
AU17 | 12 BGA-AU17 RSV164
AV16 | 13 BGA-AV16 RSV166
AV15 | 14 BGA-AV15 RSV165
AW14 | 15 BGA-AW14 RSV168
AW13 | 16 BGA-AW13 RSV167
AU13 | 17 BGA-AU13 RSV169
AU14 | 18 BGA-AU14 RSV170
AV13 | 19 BGA-AV13 RSV172
AV12 | 20 BGA-AV12 RSV171
AW11 | 21 BGA-AW11 HYP0RXP0
AP17 | 22 BGA-AP17 RSV173
AP18 | 23 BGA-AP18 RSV174
AR17 | 24 BGA-AR17 RSV176
AR16 | 25 BGA-AR16 RSV175
AT16 | 26 BGA-AT16 RSV178
AT15 | 27 BGA-AT15 RSV177
AP14 | 28 BGA-AP14 RSV179
AP15 | 29 BGA-AP15 RSV180
AR14 | 30 BGA-AR14 RSV182
AR13 | 31 BGA-AR13 RSV181
AT13 | 32 BGA-AT13 RSV184
AT12 | 33 BGA-AT12 RSV183
AL2  | 34 BGA-AL2 ALTCORECLKN
AM2  | 35 BGA-AM2 ALTCORECLKP
AM4  | 36 BGA-AM4 RSV003
AF5  | 37 BGA-AF5 BOOTCOMPLETE
AG2  | 38 BGA-AG2 HYP1RXFLDAT
AG3  | 39 BGA-AG3 HYP0RXPMDAT
AL4  | 40 BGA-AL4 CORECLKSEL
AK5  | 41 BGA-AK5 RSV012
AK1  | 42 BGA-AK1 SYSCLKOUT
AN4  | 43 BGA-AN4 RSV002
F24  | 44 BGA-F24 CORESEL0
E24  | 45 BGA-E24 CORESEL1
G24  | 46 BGA-G24 CORESEL3
D24  | 47 BGA-D24 CORESEL2
D25  | 48 BGA-D25 SPI2CLK
E8   | 49 BGA-E8 DDR3AA00
F8   | 50 BGA-F8 DDR3AA05
F9   | 51 BGA-F9 DDR3AA04
G9   | 52 BGA-G9 DDR3AA01
G8   | 53 BGA-G8 DDR3AA02
A6   | 54 BGA-A6 DDR3ADQM2
G10  | 55 BGA-G10 DDR3AA03
D8   | 56 BGA-D8 DDR3AA09
C9   | 57 BGA-C9 DDR3AA06
B9   | 58 BGA-B9 DDR3AA08
D9   | 59 BGA-D9 DDR3AA07
A9   | 60 BGA-A9 DDR3AA11
F10  | 61 BGA-F10 DDR3AA10
E10  | 62 BGA-E10 DDR3AA12
D10  | 63 BGA-D10 DDR3AA15
A10  | 64 BGA-A10 DDR3AA13
B10  | 65 BGA-B10 DDR3AA14
F13  | 66 BGA-F13 RSV029
G13  | 67 BGA-G13 DDR3AODT1
D13  | 68 BGA-D13 RSV028
B11  | 69 BGA-B11 DDR3ABA0
C11  | 70 BGA-C11 DDR3ABA1
G12  | 71 BGA-G12 DDR3ACKE0
D11  | 72 BGA-D11 DDR3ACE0
G11  | 73 BGA-G11 DDR3ABA2
F11  | 74 BGA-F11 DDR3ACE1
H10  | 75 BGA-H10 DDR3ARZQ1
C13  | 76 BGA-C13 DDR3ACAS
A11  | 77 BGA-A11 DDR3ACKE1
A16  | 78 BGA-A16 DDR3ACB00
B16  | 79 BGA-B16 DDR3ACB02
C15  | 80 BGA-C15 DDR3ACB01
D15  | 81 BGA-D15 DDR3ACB04
F15  | 82 BGA-F15 DDR3ACB03
F14  | 83 BGA-F14 DDR3ACB05
E14  | 84 BGA-E14 DDR3ADQM8
D14  | 85 BGA-D14 DDR3ACB06
G15  | 86 BGA-G15 DDR3ACB07
F12  | 87 BGA-F12 DDR3AWE
D12  | 88 BGA-D12 RSV027
A25  | 89 BGA-A25 DDR3ACLKN
B25  | 90 BGA-B25 DDR3ACLKP
B24  | 91 BGA-B24 RSV004
B12  | 92 BGA-B12 DDR3ACLKOUTN0
A12  | 93 BGA-A12 DDR3ACLKOUTP0
B13  | 94 BGA-B13 DDR3ACLKOUTN1
A13  | 95 BGA-A13 DDR3ACLKOUTP1
G1   | 96 BGA-G1 DDR3AD00
H2   | 97 BGA-H2 DDR3AD01
G2   | 98 BGA-G2 DDR3AD03
H1   | 99 BGA-H1 DDR3AD04
F1   | 100 BGA-F1 DDR3AD02
E1   | 101 BGA-E1 DDR3ADQS0P
E2   | 102 BGA-E2 DDR3AD05
D2   | 103 BGA-D2 DDR3AD07
F2   | 104 BGA-F2 DDR3AD06
D1   | 105 BGA-D1 DDR3ADQS0N
C2   | 106 BGA-C2 DDR3ADQM0
E4   | 107 BGA-E4 DDR3AD08
D4   | 108 BGA-D4 DDR3AD15
D3   | 109 BGA-D3 DDR3AD14
F4   | 110 BGA-F4 DDR3AD09
G3   | 111 BGA-G3 DDR3AD10
F3   | 112 BGA-F3 DDR3ADQM1
H3   | 113 BGA-H3 DDR3AD13
A4   | 114 BGA-A4 DDR3AD11
B4   | 115 BGA-B4 DDR3AD12
G4   | 116 BGA-G4 DDR3AD16
H5   | 117 BGA-H5 DDR3AD17
G5   | 118 BGA-G5 DDR3AD20
D5   | 119 BGA-D5 DDR3AD18
F5   | 120 BGA-F5 DDR3AD19
A5   | 121 BGA-A5 DDR3ADQS2P
D6   | 122 BGA-D6 DDR3AD21
B6   | 123 BGA-B6 DDR3AD23
C5   | 124 BGA-C5 DDR3AD22
B5   | 125 BGA-B5 DDR3ADQS2N
C7   | 126 BGA-C7 DDR3AD24
D7   | 127 BGA-D7 DDR3AD31
B8   | 128 BGA-B8 DDR3AD28
F7   | 129 BGA-F7 DDR3AD25
G7   | 130 BGA-G7 DDR3AD30
F6   | 131 BGA-F6 DDR3AD26
E6   | 132 BGA-E6 DDR3ADQM3
G6   | 133 BGA-G6 DDR3AD29
A8   | 134 BGA-A8 DDR3AD27
B7   | 135 BGA-B7 DDR3ADQS3P
E16  | 136 BGA-E16 DDR3AD32
D16  | 137 BGA-D16 DDR3AD36
F16  | 138 BGA-F16 DDR3AD34
G16  | 139 BGA-G16 DDR3AD33
G17  | 140 BGA-G17 DDR3AD35
F17  | 141 BGA-F17 DDR3AD38
H16  | 142 BGA-H16 DDR3ARZQ0
D17  | 143 BGA-D17 DDR3AD37
C17  | 144 BGA-C17 DDR3ADQM4
E18  | 145 BGA-E18 DDR3AD39
A20  | 146 BGA-A20 DDR3AD48
C19  | 147 BGA-C19 DDR3AD40
D19  | 148 BGA-D19 DDR3AD41
F19  | 149 BGA-F19 DDR3AD43
G18  | 150 BGA-G18 DDR3AD42
F18  | 151 BGA-F18 DDR3AD47
A19  | 152 BGA-A19 DDR3ADQS5N
G19  | 153 BGA-G19 DDR3AD44
B19  | 154 BGA-B19 DDR3ADQS5P
B18  | 155 BGA-B18 DDR3AD45
A18  | 156 BGA-A18 DDR3ADQM5
D18  | 157 BGA-D18 DDR3AD46
B20  | 158 BGA-B20 DDR3AD49
D20  | 159 BGA-D20 DDR3AD50
G20  | 160 BGA-G20 DDR3AD51
F20  | 161 BGA-F20 DDR3AD54
C21  | 162 BGA-C21 DDR3AD52
D21  | 163 BGA-D21 DDR3ADQM6
G21  | 164 BGA-G21 DDR3AD55
E20  | 165 BGA-E20 DDR3AD53
H22  | 166 BGA-H22 DDR3ARZQ2
C23  | 167 BGA-C23 DDR3AD56
D23  | 168 BGA-D23 DDR3AD58
G22  | 169 BGA-G22 DDR3AD57
A24  | 170 BGA-A24 RSV005
F22  | 171 BGA-F22 DDR3AD59
E22  | 172 BGA-E22 DDR3AD60
A23  | 173 BGA-A23 DDR3ADQS7P
F21  | 174 BGA-F21 DDR3AD62
B22  | 175 BGA-B22 DDR3AD61
D22  | 176 BGA-D22 DDR3AD63
A22  | 177 BGA-A22 DDR3ADQM7
A7   | 178 BGA-A7 DDR3ADQS3N
C3   | 179 BGA-C3 DDR3ADQS1N
B3   | 180 BGA-B3 DDR3ADQS1P
B17  | 181 BGA-B17 DDR3ADQS4N
A17  | 182 BGA-A17 DDR3ADQS4P
B21  | 183 BGA-B21 DDR3ADQS6N
A21  | 184 BGA-A21 DDR3ADQS6P
B23  | 185 BGA-B23 DDR3ADQS7N
A15  | 186 BGA-A15 DDR3ADQS8N
B15  | 187 BGA-B15 DDR3ADQS8P
E12  | 188 BGA-E12 DDR3AODT0
A14  | 189 BGA-A14 DDR3ARAS
B14  | 190 BGA-B14 DDR3ARESET
AA32 | 191 BGA-AA32 DDR3BA00
W34  | 192 BGA-W34 DDR3BA04
V34  | 193 BGA-V34 DDR3BA05
W33  | 194 BGA-W33 DDR3BA01
Y32  | 195 BGA-Y32 DDR3BA09
W32  | 196 BGA-W32 DDR3BA02
U39  | 197 BGA-U39 DDR3BDQM2
Y34  | 198 BGA-Y34 DDR3BA03
AA33 | 199 BGA-AA33 DDR3BA08
W36  | 200 BGA-W36 DDR3BA06
Y35  | 201 BGA-Y35 DDR3BA12
W37  | 202 BGA-W37 DDR3BA07
Y36  | 203 BGA-Y36 DDR3BA15
Y38  | 204 BGA-Y38 DDR3BA10
Y39  | 205 BGA-Y39 DDR3BA13
AA39 | 206 BGA-AA39 DDR3BA11
AA38 | 207 BGA-AA38 DDR3BA14
AB32 | 208 BGA-AB32 RSV032
AC32 | 209 BGA-AC32 DDR3BRESET
AC33 | 210 BGA-AC33 DDR3BODT0
AA37 | 211 BGA-AA37 DDR3BBA0
AA36 | 212 BGA-AA36 DDR3BCE1
AA31 | 213 BGA-AA31 DDR3BRZQ0
AA34 | 214 BGA-AA34 DDR3BBA1
AB35 | 215 BGA-AB35 DDR3BBA2
AB34 | 216 BGA-AB34 DDR3BCE0
AC36 | 217 BGA-AC36 DDR3BCAS
AC37 | 218 BGA-AC37 DDR3BWE
AD35 | 219 BGA-AD35 RSV030
AF32 | 220 BGA-AF32 DDR3BCB00
AE32 | 221 BGA-AE32 DDR3BCB02
AF34 | 222 BGA-AF34 DDR3BCB01
AE33 | 223 BGA-AE33 DDR3BCB04
AF35 | 224 BGA-AF35 DDR3BCB03
AE36 | 225 BGA-AE36 DDR3BCB05
AD36 | 226 BGA-AD36 DDR3BCB06
AE34 | 227 BGA-AE34 DDR3BCB07
AE37 | 228 BGA-AE37 DDR3BDQM8
AB38 | 229 BGA-AB38 DDR3BCKE1
AB39 | 230 BGA-AB39 DDR3BCKE0
AR39 | 231 BGA-AR39 DDR3BCLKN
AR38 | 232 BGA-AR38 DDR3BCLKP
AP38 | 233 BGA-AP38 RSV006
AD39 | 234 BGA-AD39 DDR3BCLKOUTN0
AD38 | 235 BGA-AD38 DDR3BCLKOUTP0
AD32 | 236 BGA-AD32 DDR3BRAS
AC38 | 237 BGA-AC38 DDR3BCLKOUTN1
AC39 | 238 BGA-AC39 DDR3BCLKOUTP1
AC34 | 239 BGA-AC34 RSV031
L38  | 240 BGA-L38 DDR3BD00
L39  | 241 BGA-L39 DDR3BD03
N34  | 242 BGA-N34 DDR3BD01
N33  | 243 BGA-N33 DDR3BD04
M37  | 244 BGA-M37 DDR3BD02
M38  | 245 BGA-M38 DDR3BDQS0P
M36  | 246 BGA-M36 EMIFD14
N37  | 247 BGA-N37 DDR3BD05
N38  | 248 BGA-N38 DDR3BD07
N36  | 249 BGA-N36 DDR3BD06
N39  | 250 BGA-N39 DDR3BDQM0
T32  | 251 BGA-T32 DDR3BD08
R33  | 252 BGA-R33 DDR3BD14
P36  | 253 BGA-P36 DDR3BD15
R32  | 254 BGA-R32 DDR3BD09
P35  | 255 BGA-P35 DDR3BD10
N32  | 256 BGA-N32 DDR3BD13
P32  | 257 BGA-P32 DDR3BRZQ1
R39  | 258 BGA-R39 DDR3BD11
R38  | 259 BGA-R38 DDR3BD12
U32  | 260 BGA-U32 DDR3BDQM3
T34  | 261 BGA-T34 DDR3BD16
R36  | 262 BGA-R36 DDR3BD20
R34  | 263 BGA-R34 DDR3BD17
T35  | 264 BGA-T35 DDR3BD18
R37  | 265 BGA-R37 DDR3BD19
U37  | 266 BGA-U37 DDR3BD21
T36  | 267 BGA-T36 DDR3BD22
U38  | 268 BGA-U38 DDR3BD23
T38  | 269 BGA-T38 DDR3BDQS2N
V35  | 270 BGA-V35 DDR3BD24
V36  | 271 BGA-V36 DDR3BD31
U36  | 272 BGA-U36 DDR3BD25
V32  | 273 BGA-V32 DDR3BD30
U34  | 274 BGA-U34 DDR3BD26
U33  | 275 BGA-U33 DDR3BD29
W38  | 276 BGA-W38 DDR3BD27
W39  | 277 BGA-W39 DDR3BD28
AG37 | 278 BGA-AG37 DDR3BD32
AF36 | 279 BGA-AF36 DDR3BD33
AG36 | 280 BGA-AG36 DDR3BD36
AG38 | 281 BGA-AG38 DDR3BD34
AG34 | 282 BGA-AG34 DDR3BD35
AH35 | 283 BGA-AH35 DDR3BD38
AH34 | 284 BGA-AH34 DDR3BD37
AG33 | 285 BGA-AG33 DDR3BDQM4
AG32 | 286 BGA-AG32 DDR3BD39
AH32 | 287 BGA-AH32 DDR3BD40
AJ33 | 288 BGA-AJ33 DDR3BD41
AJ34 | 289 BGA-AJ34 DDR3BD43
AH36 | 290 BGA-AH36 DDR3BD42
AJ37 | 291 BGA-AJ37 DDR3BD47
AJ38 | 292 BGA-AJ38 DDR3BDQS5N
AJ36 | 293 BGA-AJ36 DDR3BD44
AH39 | 294 BGA-AH39 DDR3BD45
AG39 | 295 BGA-AG39 DDR3BDQM5
AH38 | 296 BGA-AH38 DDR3BD46
AK39 | 297 BGA-AK39 DDR3BD48
AK38 | 298 BGA-AK38 DDR3BD49
AL39 | 299 BGA-AL39 DDR3BDQS6P
AK36 | 300 BGA-AK36 DDR3BD50
AK35 | 301 BGA-AK35 DDR3BD51
AL37 | 302 BGA-AL37 DDR3BD54
AL34 | 303 BGA-AL34 DDR3BD52
AL33 | 304 BGA-AL33 DDR3BD55
AK32 | 305 BGA-AK32 DDR3BRZQ2
AL36 | 306 BGA-AL36 DDR3BD53
AK34 | 307 BGA-AK34 DDR3BDQM6
AN34 | 308 BGA-AN34 DDR3BD56
AN36 | 309 BGA-AN36 DDR3BD57
AN33 | 310 BGA-AN33 DDR3BD58
AN39 | 311 BGA-AN39 DDR3BDQS7N
AP39 | 312 BGA-AP39 RSV007
AM34 | 313 BGA-AM34 DDR3BD59
AM35 | 314 BGA-AM35 DDR3BD60
AM36 | 315 BGA-AM36 DDR3BD62
AM38 | 316 BGA-AM38 DDR3BD61
AM39 | 317 BGA-AM39 DDR3BDQM7
AN37 | 318 BGA-AN37 DDR3BD63
P34  | 319 BGA-P34 DDR3BDQM1
P38  | 320 BGA-P38 DDR3BDQS1N
M39  | 321 BGA-M39 DDR3BDQS0N
P39  | 322 BGA-P39 DDR3BDQS1P
T39  | 323 BGA-T39 DDR3BDQS2P
V38  | 324 BGA-V38 DDR3BDQS3N
V39  | 325 BGA-V39 DDR3BDQS3P
AF39 | 326 BGA-AF39 DDR3BDQS4N
AF38 | 327 BGA-AF38 DDR3BDQS4P
AJ39 | 328 BGA-AJ39 DDR3BDQS5P
AL38 | 329 BGA-AL38 DDR3BDQS6N
AN38 | 330 BGA-AN38 DDR3BDQS7P
AE38 | 331 BGA-AE38 DDR3BDQS8N
AE39 | 332 BGA-AE39 DDR3BDQS8P
AD34 | 333 BGA-AD34 DDR3BODT1
P2   | 334 BGA-P2 RSV000
P1   | 335 BGA-P1 RSV001
R4   | 336 BGA-R4 EMU17
F34  | 337 BGA-F34 EMIFA00
E34  | 338 BGA-E34 EMIFA04
C35  | 339 BGA-C35 EMIFA08
F37  | 340 BGA-F37 EMIFA01
E38  | 341 BGA-E38 EMIFWAIT0
G36  | 342 BGA-G36 EMIFA02
E39  | 343 BGA-E39 EMIFA03
H35  | 344 BGA-H35 EMIFA06
H33  | 345 BGA-H33 EMIFBE1
J34  | 346 BGA-J34 EMIFA05
K33  | 347 BGA-K33 EMIFA07
F38  | 348 BGA-F38 EMIFA10
D35  | 349 BGA-D35 EMIFA11
G37  | 350 BGA-G37 EMIFA09
H36  | 351 BGA-H36 EMIFA12
E35  | 352 BGA-E35 EMIFA13
F39  | 353 BGA-F39 EMIFA15
F35  | 354 BGA-F35 EMIFA17
G38  | 355 BGA-G38 EMIFA14
J35  | 356 BGA-J35 EMIFA18
K34  | 357 BGA-K34 EMIFA16
J36  | 358 BGA-J36 EMIFA21
C36  | 359 BGA-C36 EMIFA20
G39  | 360 BGA-G39 EMIFA19
H38  | 361 BGA-H38 EMIFA22
D36  | 362 BGA-D36 EMIFA23
M32  | 363 BGA-M32 EMIFD00
H34  | 364 BGA-H34 EMIFBE0
D39  | 365 BGA-D39 EMIFWAIT1
F36  | 366 BGA-F36 EMIFWE
G33  | 367 BGA-G33 EMIFCE0
F33  | 368 BGA-F33 EMIFRNW
G32  | 369 BGA-G32 EMIFCE1
B36  | 370 BGA-B36 GPIO30
G34  | 371 BGA-G34 EMIFCE2
E36  | 372 BGA-E36 EMIFCE3
E33  | 373 BGA-E33 RSV015
E37  | 374 BGA-E37 EMIFOE
L33  | 375 BGA-L33 EMIFD02
J37  | 376 BGA-J37 EMIFD01
H39  | 377 BGA-H39 EMIFD04
L34  | 378 BGA-L34 EMIFD03
J38  | 379 BGA-J38 EMIFD05
J39  | 380 BGA-J39 EMIFD07
K37  | 381 BGA-K37 EMIFD06
K38  | 382 BGA-K38 EMIFD09
K36  | 383 BGA-K36 EMIFD10
K39  | 384 BGA-K39 EMIFD08
L35  | 385 BGA-L35 EMIFD12
L36  | 386 BGA-L36 EMIFD11
M34  | 387 BGA-M34 EMIFD13
M35  | 388 BGA-M35 EMIFD15
AA2  | 389 BGA-AA2 EMU00
Y3   | 390 BGA-Y3 EMU02
AB1  | 391 BGA-AB1 TSCOMPOUT
AB2  | 392 BGA-AB2 EMU01
AB3  | 393 BGA-AB3 EMU14
AC4  | 394 BGA-AC4 RSV188
Y4   | 395 BGA-Y4 EMU03
W3   | 396 BGA-W3 EMU04
W4   | 397 BGA-W4 EMU05
V4   | 398 BGA-V4 EMU06
U3   | 399 BGA-U3 EMU08
U4   | 400 BGA-U4 EMU07
T3   | 401 BGA-T3 EMU09
U5   | 402 BGA-U5 EMU12
AB4  | 403 BGA-AB4 EMU10
AA3  | 404 BGA-AA3 EMU11
AA4  | 405 BGA-AA4 EMU18
T4   | 406 BGA-T4 EMU13
R3   | 407 BGA-R3 EMU15
T5   | 408 BGA-T5 EMU16
AC3  | 409 BGA-AC3 TSSYNCEVT
F29  | 410 BGA-F29 GPIO00
E29  | 411 BGA-E29 GPIO05
A30  | 412 BGA-A30 GPIO08
B30  | 413 BGA-B30 GPIO01
C30  | 414 BGA-C30 GPIO07
D29  | 415 BGA-D29 GPIO02
B29  | 416 BGA-B29 GPIO04
A35  | 417 BGA-A35 GPIO03
A36  | 418 BGA-A36 GPIO16
G30  | 419 BGA-G30 GPIO09
D30  | 420 BGA-D30 GPIO06
E30  | 421 BGA-E30 GPIO11
F31  | 422 BGA-F31 GPIO10
E32  | 423 BGA-E32 GPIO14
F30  | 424 BGA-F30 GPIO12
A31  | 425 BGA-A31 GPIO13
B31  | 426 BGA-B31 GPIO15
D33  | 427 BGA-D33 GPIO21
A32  | 428 BGA-A32 GPIO17
C31  | 429 BGA-C31 GPIO18
B32  | 430 BGA-B32 GPIO19
A33  | 431 BGA-A33 GPIO20
D31  | 432 BGA-D31 GPIO22
C34  | 433 BGA-C34 GPIO29
B33  | 434 BGA-B33 GPIO24
B35  | 435 BGA-B35 GPIO23
A34  | 436 BGA-A34 GPIO26
E31  | 437 BGA-E31 GPIO25
D32  | 438 BGA-D32 GPIO27
C33  | 439 BGA-C33 GPIO28
B34  | 440 BGA-B34 GPIO31
AE5  | 441 BGA-AE5 HOUT
AE4  | 442 BGA-AE4 LRESET
AE1  | 443 BGA-AE1 TCK
AD4  | 444 BGA-AD4 LRESETNMIEN
AD3  | 445 BGA-AD3 RESETFULL
AD5  | 446 BGA-AD5 NMI
AT10 | 447 BGA-AT10 HYP0CLKN
AT9  | 448 BGA-AT9 HYP0CLKP
AU10 | 449 BGA-AU10 HYP0RXN1
AM7  | 450 BGA-AM7 RSV020
AJ5  | 451 BGA-AJ5 HYP0RXFLCLK
AK4  | 452 BGA-AK4 POR
AJ4  | 453 BGA-AJ4 HYP0RXFLDAT
AJ3  | 454 BGA-AJ3 HYP0TXFLCLK
AW10 | 455 BGA-AW10 HYP0RXN0
AU11 | 456 BGA-AU11 HYP0RXP1
AV9  | 457 BGA-AV9 HYP0RXN2
AV10 | 458 BGA-AV10 HYP0RXP2
AW8  | 459 BGA-AW8 HYP0RXP3
AW7  | 460 BGA-AW7 HYP0RXN3
AJ2  | 461 BGA-AJ2 HYP0RXPMCLK
AJ1  | 462 BGA-AJ1 HYP0TXPMDAT
AG5  | 463 BGA-AG5 HYP0TXFLDAT
AP11 | 464 BGA-AP11 HYP0TXN0
AP12 | 465 BGA-AP12 HYP0TXP0
AR11 | 466 BGA-AR11 HYP0TXP1
AR10 | 467 BGA-AR10 HYP0TXN1
AP9  | 468 BGA-AP9 HYP0TXP2
AP8  | 469 BGA-AP8 HYP0TXN2
AR8  | 470 BGA-AR8 HYP0TXP3
AR7  | 471 BGA-AR7 HYP0TXN3
AT7  | 472 BGA-AT7 HYP1TXP0
AH5  | 473 BGA-AH5 HYP0TXPMCLK
AH4  | 474 BGA-AH4 HYP1RXFLCLK
AM6  | 475 BGA-AM6 HYP1REFRES
AW5  | 476 BGA-AW5 HYP1CLKN
AW4  | 477 BGA-AW4 HYP1CLKP
AV6  | 478 BGA-AV6 HYP1RXN1
AH3  | 479 BGA-AH3 HYP1TXFLCLK
AU7  | 480 BGA-AU7 HYP1RXN0
AU8  | 481 BGA-AU8 HYP1RXP0
AV7  | 482 BGA-AV7 HYP1RXP1
AU4  | 483 BGA-AU4 HYP1RXN2
AU5  | 484 BGA-AU5 HYP1RXP2
AV4  | 485 BGA-AV4 HYP1RXP3
AV3  | 486 BGA-AV3 HYP1RXN3
AF3  | 487 BGA-AF3 HYP1RXPMCLK
AG1  | 488 BGA-AG1 TDI
AF4  | 489 BGA-AF4 HYP1RXPMDAT
AH1  | 490 BGA-AH1 HYP1TXPMCLK
AH2  | 491 BGA-AH2 HYP1TXFLDAT
AT6  | 492 BGA-AT6 HYP1TXN0
AP6  | 493 BGA-AP6 HYP1TXP1
AP5  | 494 BGA-AP5 HYP1TXN1
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| Models and submodels in the file (103): PDDRIO_D3FP3_34 (I/O), PDDRIO_D3FP3_40 (I/O), PDDRIO_D3FP3_48 (I/O), PDDRIO_D3FP3_ODT120 (Input), PDDRIO_D3FP3_ODT40 (Input), PDDRIO_D3FP3_ODT60 (Input), PDDRIO_D3FP3_ODTOFF (Input), PDDRIO_D3FP3L_34 (I/O), PDDRIO_D3FP3L_40 (I/O), PDDRIO_D3FP3L_48 (I/O), PDDRIO_D3FP3L_ODT120 (Input), PDDRIO_D3FP3L_ODT40 (Input), PDDRIO_D3FP3L_ODT60 (Input), PDDRIO_D3FP3L_ODTOFF (Input), PDIFF_D3FF3_34 (I/O), PDIFF_D3FF3_40 (I/O), PDIFF_D3FF3_48 (I/O), PDIFF_D3FF3_ODT120 (Input), PDIFF_D3FF3_ODT40 (Input), PDIFF_D3FF3_ODT60 (Input), PDIFF_D3FF3_ODTOFF (Input), PDIFF_D3FF3L_34 (I/O), PDIFF_D3FF3L_40 (I/O), PDIFF_D3FF3L_48 (I/O), PDIFF_D3FF3L_ODT120 (Input), PDIFF_D3FF3L_ODT40 (Input), PDIFF_D3FF3L_ODT60 (Input), PDIFF_D3FF3L_ODTOFF (Input), bc181540h_40CCLASS_1P5 (I/O), bc181540h_WK_PD_ON_1P5 (Input), bc181540h_40ECLASS_1P5 (I/O), bc181540h_WK_PU_ON_1P5 (Input), bc181540h_40DCLASS_1P5 (I/O), bc181540h_50BCLASS_1P5 (I/O), bc181540h_40CCLASS_1P8 (I/O), bc181540h_WK_PD_ON_1P8 (Input), bc181540h_40ECLASS_1P8 (I/O), bc181540h_WK_PU_ON_1P8 (Input), bc181540h_40DCLASS_1P8 (I/O), bc181540h_50BCLASS_1P8 (I/O), bc181540v_40CCLASS_1P5 (I/O), bc181540v_WK_PD_ON_1P5 (Input), bc181540v_40ECLASS_1P5 (I/O), bc181540v_WK_PU_ON_1P5 (Input), bc181540v_40DCLASS_1P5 (I/O), bc181540v_50BCLASS_1P5 (I/O), bc181540v_40CCLASS_1P8 (I/O), bc181540v_WK_PD_ON_1P8 (Input), bc181540v_40ECLASS_1P8 (I/O), bc181540v_WK_PU_ON_1P8 (Input), bc181540v_40DCLASS_1P8 (I/O), bc181540v_50BCLASS_1P8 (I/O), bi2c1815h_HS_SLAVE_MODE_1P5 (I/O_open_drain), bi2c1815h_FAST_STD_1P5 (I/O_open_drain), bi2c1815h_HS_MASTER_MODE_1P5 (I/O), bi2c1815h_HS_SLAVE_MODE_1P8 (I/O_open_drain), bi2c1815h_FAST_STD_1P8 (I/O_open_drain), bi2c1815h_HS_MASTER_MODE_1P8 (I/O), bi2c1815v_HS_SLAVE_MODE_1P5 (I/O_open_drain), bi2c1815v_FAST_STD_1P5 (I/O_open_drain), bi2c1815v_HS_MASTER_MODE_1P5 (I/O), bi2c1815v_HS_SLAVE_MODE_1P8 (I/O_open_drain), bi2c1815v_FAST_STD_1P8 (I/O_open_drain), bi2c1815v_HS_MASTER_MODE_1P8 (I/O), ic1815h_WK_PD_ON_1P5 (Input), ic1815h_WK_PU_ON_1P5 (Input), ic1815h_RX_MODE_1P5 (Input), ic1815h_WK_PD_ON_1P8 (Input), ic1815h_WK_PU_ON_1P8 (Input), ic1815h_RX_MODE_1P8 (Input), ic1815v_WK_PD_ON_1P5 (Input), ic1815v_WK_PU_ON_1P5 (Input), ic1815v_RX_MODE_1P5 (Input), ic1815v_WK_PD_ON_1P8 (Input), ic1815v_WK_PU_ON_1P8 (Input), ic1815v_RX_MODE_1P8 (Input), iclkrx0p9gh_encmint_0 (Input), s_iclkrx0p9gh_encmint_0 (Series), iclkrx0p9gh_encmint_1 (Input), s_iclkrx0p9gh_encmint_1 (Series)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
